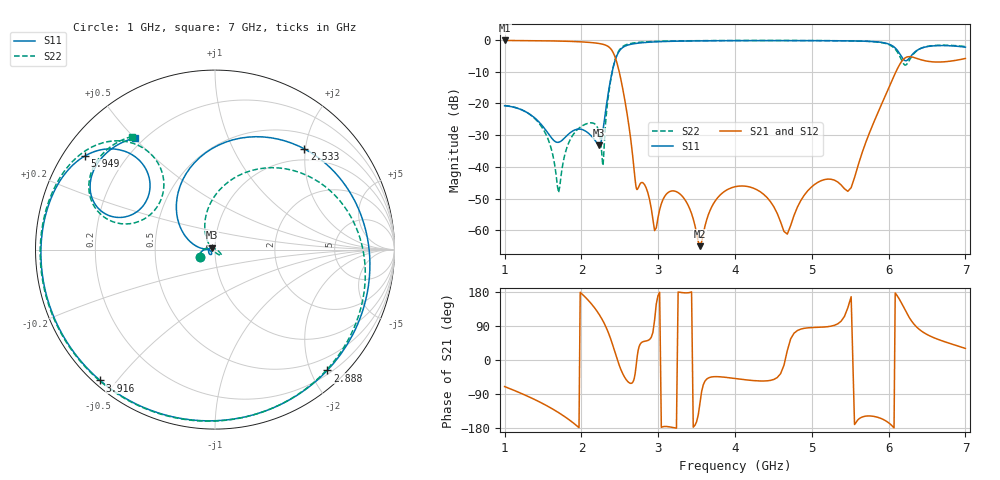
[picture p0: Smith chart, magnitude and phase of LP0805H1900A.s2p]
! Created Mon Mar 25 10:21:34 2019
! AVX THIN FILM OPERATION
! LP0805 High Performance Low Pass Filter P/N  LP0805H1900ASTR
! List of port names and net name(s): example Port n = <port_name> <net_name1> <net_name2> ...
! Port 1 = P1 N__9
! Port 2 = P2 N__12
# mhz S db R 50
! 2 Port Network Data from data block
! freq  dbS11  angS11  dbS21  angS21  dbS12  angS12  dbS22  angS22
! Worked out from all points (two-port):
!   449 points, 1 GHz to 7 GHz, reference 50 ohm
!   highest |S21| = -0.20 dB at 1 GHz (marker M1); lowest = -65.0 dB at 3.544 GHz (marker M2)
!   |S21| within 3 dB of the highest: start of sweep to 2.394 GHz
!   lowest |S11| = -33.3 dB at 2.233 GHz (marker M3), VSWR 1.04, Z = 48.2 + j1.1 ohm
!   |S11| at or under -10 dB: start of sweep to 2.401 GHz
!   |S22| runs from -48.1 to -0.2 dB; largest |S21 - S12| = 0
!   S11 on the Smith chart (normalised r, x): 1 GHz: 0.85, -0.07; 2.533 GHz: 0.77, +1.98; 2.888 GHz: 0.26, -2.27; 3.916 GHz: 0.02, -0.45; 5.949 GHz: 0.06, +0.32; 7 GHz: 0.17, +0.50
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1000  -20.75 -153.9  -0.20 -70.1  -0.20 -70.1  -20.70 -152.4
1476.562  -26.62 179.2  -0.30 -112.9  -0.30 -112.9  -27.18 167.8
1703.125  -32.26 -145.1  -0.39 -138.9  -0.39 -138.9  -48.11 64.7
2000  -28.18 -150.3  -0.64 175.7  -0.64 175.7  -27.24 -37.0
2233.333  -33.26 148.4  -1.17 119.6  -1.17 119.6  -29.47 -54.6
2283.333  -28.10 175.5  -1.42 102.1  -1.42 102.1  -39.07 -157.8
2383.333  -12.10 144.2  -2.86 54.3  -2.86 54.3  -12.41 98.5
2533.333  -2.50 48.4  -14.79 -34.1  -14.79 -34.1  -2.18 13.8
2716.667  -1.11 -14.6  -46.83 -7.8  -46.83 -7.8  -0.87 -39.5
2887.5  -0.73 -47.1  -50.28 54.0  -50.28 54.0  -0.57 -66.7
3018.75  -0.58 -65.0  -53.47 178.6  -53.47 178.6  -0.45 -81.8
3259.375  -0.42 -89.4  -48.10 179.4  -48.10 179.4  -0.33 -102.7
3543.75  -0.32 -110.5  -64.96 -113.6  -64.96 -113.6  -0.26 -121.2
3915.625  -0.26 -131.3  -46.97 -46.6  -46.97 -46.6  -0.22 -139.9
4003.125  -0.26 -135.5  -46.23 -48.9  -46.23 -48.9  -0.22 -143.7
4681.25  -0.24 -163.2  -61.16 25.0  -61.16 25.0  -0.21 -169.4
5031.25  -0.26 -175.7  -45.62 85.9  -45.62 85.9  -0.23 178.8
5512.5  -0.34 166.8  -46.54 167.0  -46.54 167.0  -0.33 161.9
5949.392  -0.97 144.4  -18.02 -158.9  -18.02 -158.9  -1.08 138.9
6010.156  -1.41 139.4  -14.66 -167.2  -14.66 -167.2  -1.58 133.5
6298.785  -4.89 161.7  -5.37 103.0  -5.37 103.0  -5.31 164.6
7000  -2.31 125.8  -5.87 30.5  -5.87 30.5  -2.13 126.3
